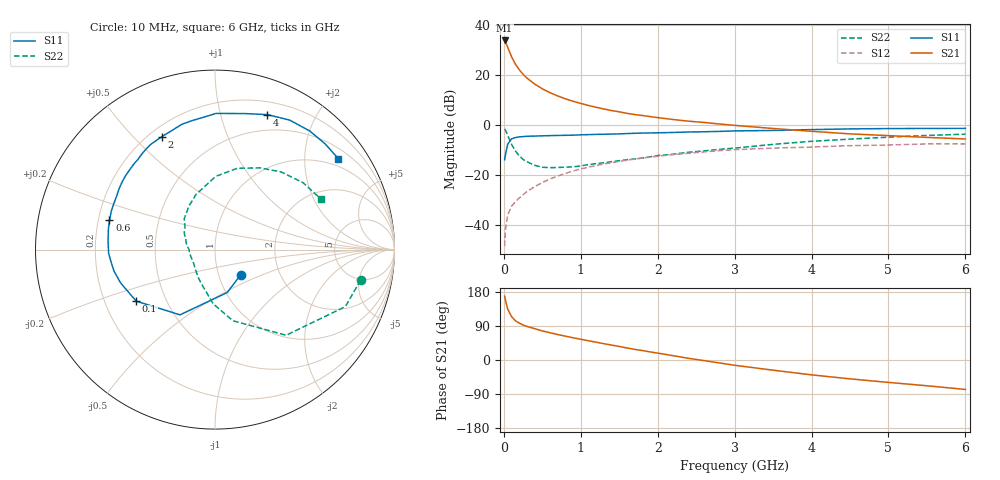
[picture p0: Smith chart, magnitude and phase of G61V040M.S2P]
! SIEMENS Small Signal Semiconductors
! BFG193
! Si NPN RF Bipolar Junction Transistor in SOT223
! VCE = 1 V  IC = 40 mA
! Common Emitter S-Parameters:  August  1996
# GHz  S  MA  R  50
!  f  S11  S21  S12  S22
! GHz  MAG  ANG  MAG  ANG  MAG  ANG  MAG  ANG
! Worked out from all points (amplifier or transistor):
!   36 points, 10 MHz to 6 GHz, reference 50 ohm
!   highest |S21| = 33.9 dB at 10 MHz (marker M1)
!   |S21| within 3 dB of that: start of sweep to 53.84 MHz
!   unconditionally stable (mu >= 1): 334.2 MHz to 4.024 GHz
!   at 250 MHz: K = 0.95, MSG = 24.1 dB, |S12| = -28.0 dB
!   at 1.4 GHz: K = 1.09, MAG = 8.6 dB, |S12| = -15.2 dB
!   at 6 GHz: K = 0.99, MSG = 1.0 dB, |S12| = -7.6 dB
!   S11 on the Smith chart (normalised r, x): 10 MHz: 1.27, -0.37; 100 MHz: 0.34, -0.27; 600 MHz: 0.25, +0.13; 2 GHz: 0.25, +0.61; 4 GHz: 0.33, +1.41; 6 GHz: 0.77, +2.87
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0.01  0.2004 -44.7  49.53 168.4  0.0037 82.1  0.8288 -11.8
0.02  0.2486 -74.0  46.77 158.6  0.0076 74.4  0.7929 -23.6
0.05  0.4124 -118.2  36.26 134.4  0.0156 62.1  0.6204 -50.3
0.1  0.5245 -146.8  23.42 114.7  0.0234 56.0  0.4087 -75.9
0.15  0.5582 -160.7  16.59 103.5  0.0289 58.0  0.3013 -92.1
0.2  0.5754 -168.1  12.84 97.4  0.0343 60.4  0.2409 -101.7
0.25  0.5838 -173.6  10.38 92.4  0.04 61.4  0.2031 -112.4
0.3  0.593 -178.0  8.735 88.7  0.046 62.7  0.1829 -120.2
0.4  0.598 175.2  6.622 82.7  0.0579 63.6  0.1552 -134.9
0.5  0.6046 169.3  5.309 76.8  0.0697 62.9  0.1418 -146.6
0.6  0.6105 164.4  4.438 72.0  0.0827 62.3  0.1388 -155.5
0.8  0.6193 155.6  3.341 62.9  0.1064 58.8  0.1425 -172.5
1.1  0.64 144.0  2.457 50.8  0.142 53.4  0.1599 170.5
1.6  0.6717 127.1  1.71 31.7  0.1963 41.5  0.2004 148.4
2  0.6956 115.2  1.402 18.2  0.2353 31.8  0.2431 134.7
2.2  0.7061 109.7  1.285 11.4  0.2537 26.9  0.2586 128.1
2.8  0.742 94.3  1.045 -7.7  0.3052 12.1  0.324 109.3
3.5  0.7755 77.8  0.849 -26.9  0.3429 -5.8  0.4079 89.5
4  0.8067 68.8  0.746 -39.2  0.3602 -15.4  0.4698 74.7
4.5  0.8329 60.0  0.662 -49.8  0.3841 -25.3  0.5198 61.2
5.5  0.8507 43.9  0.563 -68.0  0.4166 -47.7  0.616 37.3
6  0.8537 36.3  0.523 -77.7  0.4154 -60.4  0.6532 25.7
